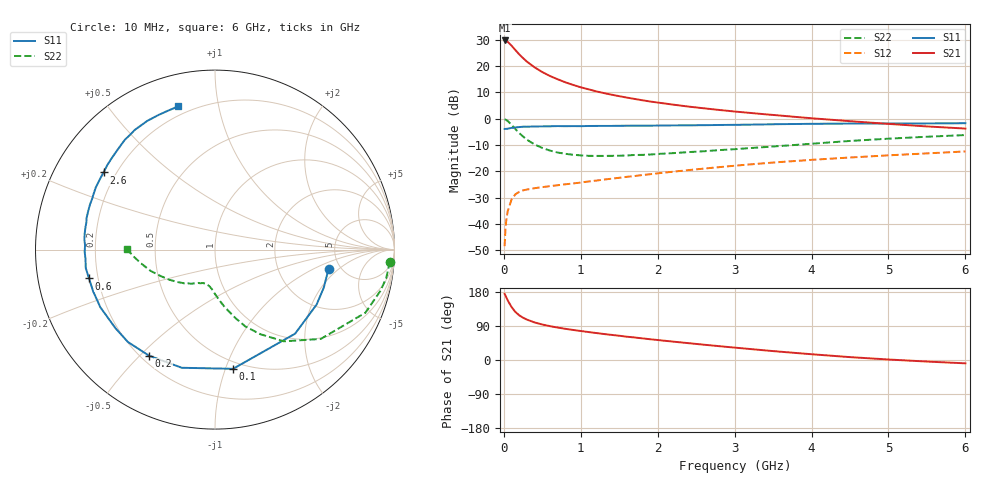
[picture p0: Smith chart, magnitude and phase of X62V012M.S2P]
! SIEMENS Small Signal Semiconductors
! BFP193W
! Si NPN RF Bipolar Junction Transistor in SOT343
! VCE = 2 V  IC = 12 mA
! Common Emitter S-Parameters:  April 1994
# GHz  S  MA  R  50
!  f  S11  S21  S12  S22
! GHz  MAG  ANG  MAG  ANG  MAG  ANG  MAG  ANG
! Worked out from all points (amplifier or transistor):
!   40 points, 10 MHz to 6 GHz, reference 50 ohm
!   highest |S21| = 29.8 dB at 10 MHz (marker M1)
!   |S21| within 3 dB of that: start of sweep to 131.1 MHz
!   unconditionally stable (mu >= 1): 1.175 GHz to 4.143 GHz
!   at 200 MHz: K = 0.26, MSG = 26.1 dB, |S12| = -27.8 dB
!   at 1.5 GHz: K = 1.09, MAG = 13.7 dB, |S12| = -22.4 dB
!   at 6 GHz: K = 0.93, MSG = 4.3 dB, |S12| = -12.4 dB
!   S11 on the Smith chart (normalised r, x): 10 MHz: 4.01, -1.48; 100 MHz: 0.44, -1.06; 200 MHz: 0.23, -0.53; 600 MHz: 0.16, -0.11; 2.6 GHz: 0.15, +0.31; 6 GHz: 0.15, +0.77
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0.01  0.6419 -9.7  30.79 174.5  0.0038 88.4  0.977 -3.9
0.02  0.642 -19.3  30.77 170.6  0.0076 80.3  0.967 -9.5
0.03  0.6436 -28.4  30.3 166.2  0.0112 78.4  0.95 -14.0
0.05  0.647 -46.4  28.98 157.5  0.0175 70.1  0.9085 -22.8
0.1  0.6718 -81.4  24.56 139.8  0.0294 55.8  0.7713 -40.2
0.15  0.6839 -105.7  20.27 126.8  0.0367 45.9  0.639 -53.1
0.2  0.696 -121.9  16.77 117.9  0.0409 40.4  0.535 -61.8
0.25  0.7073 -133.3  14.22 111.5  0.0437 36.7  0.4607 -68.4
0.3  0.7066 -141.6  12.18 106.6  0.0453 34.6  0.4002 -73.2
0.4  0.7151 -153.3  9.479 99.1  0.048 32.7  0.3252 -80.4
0.5  0.7176 -161.1  7.722 93.6  0.0503 32.9  0.2791 -85.6
0.6  0.7202 -167.1  6.492 89.3  0.0525 33.4  0.2486 -89.8
0.8  0.7233 -175.8  4.935 82.3  0.0569 36.0  0.2161 -95.7
1.1  0.7301 175.5  3.635 73.8  0.0644 39.9  0.1979 -102.9
1.3  0.7324 170.2  3.081 68.6  0.0699 42.2  0.1972 -106.7
1.6  0.7379 163.7  2.527 61.5  0.079 44.9  0.2011 -111.7
2.2  0.7492 152.4  1.859 48.5  0.0988 47.5  0.2224 -122.1
2.6  0.7555 145.3  1.582 40.4  0.1132 47.7  0.2415 -129.1
3.2  0.7741 135.7  1.294 29.0  0.1359 46.6  0.2777 -139.5
4.5  0.8104 117.7  0.901 7.6  0.1838 40.7  0.3795 -162.0
5.5  0.8171 108.6  0.716 -4.1  0.2202 35.2  0.4558 -175.2
6  0.8238 104.3  0.652 -8.8  0.2397 32.7  0.4909 179.6
